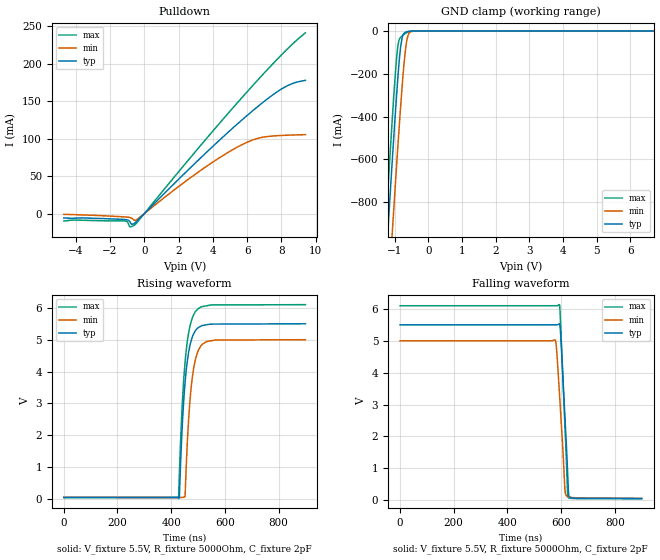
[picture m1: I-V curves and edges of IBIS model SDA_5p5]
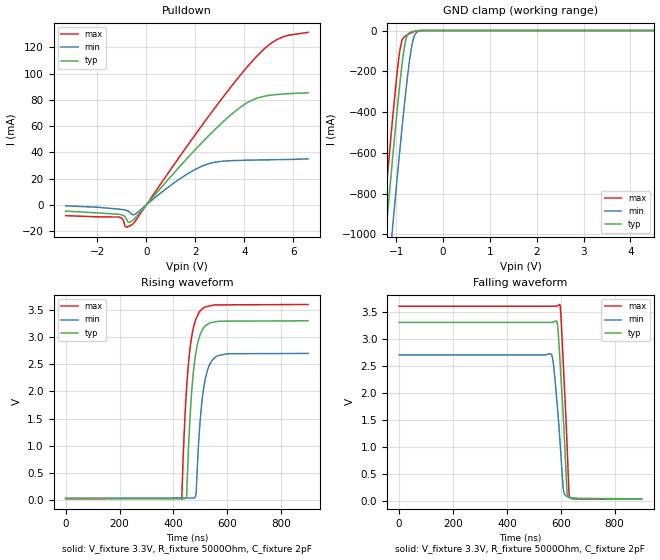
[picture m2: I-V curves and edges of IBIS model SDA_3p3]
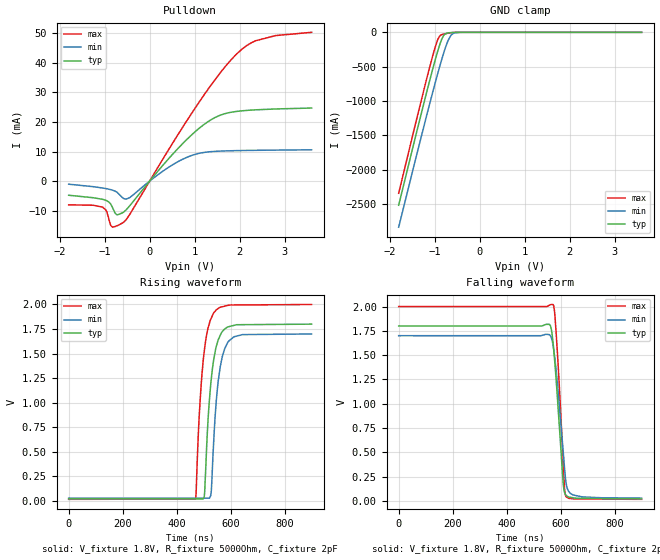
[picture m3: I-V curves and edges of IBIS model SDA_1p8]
[IBIS Ver]   4.1
[File name]   tmp4719.ibs
[File Rev]   1.0
[Date]   07/26/2024
[Source]
| Texas Instruments Incorporated.
| 12500 TI Blvd
| Dallas, TX -75243
[Notes]   Revision History:
| Rev 1.0: 07/29/2024
| - Initial version of the model
| - Model generated from simulations in TISPICE
| - C_comp although listed in numerical order of value are
|   obtained from varying PVT conditions. For PVT conditions for
|   each specific value refer the buffer description under
|   respective [Model]. IBIS model user is responsible for using
|   appropriate C_comp to simulate for Signal Integrity.
| - Warnings regarding combined Non-monotonicity of various models have been
|   reviewd and considered minor and can be ignored.
| - Model names with a trailing _1p8 contains the model for
|   1.8V operation. Model names with a trailing _3p3 contains the model
|   for 3.3V operation. Model names with a trailing _5p5 contains the model
|   for 5.5V operation.
[Disclaimer]
| This model is designed as an aid for customers of Texas Instruments.
| TI and its licensors and suppliers make no warranties, either expressed
| or implied, with respect to this  model, including the warranties of
| merchantability or fitness for a particular purpose. The model is
| provided solely on an "as is" basis. The entire risk as to its quality
| and performance is with the customer.
[Copyright]
 (C) Copyright 2024 Texas Instruments Incorporated.All rights reserved.
|   Device
[Component]   TMP4719
[Manufacturer]   TI
[Package]   |DGK 10 pin
| variable   typ   min   max
R_pkg   0.083   0.076   0.088
L_pkg   1.774nH   1.670nH   1.869nH
C_pkg   0.393pF   0.385pF   0.402pF
[Pin]  signal_name   model_name   R_pin   L_pin   C_pin
1   SDA   SDA   0.08836   1.8688nH   0.38537pF
2   SCL   SCL   0.0798   1.72452nH   0.40219pF
3   ALERT   ALERT   0.07626   1.67019nH   0.40077pF
4   T_CRIT   T_CRIT   0.07626   1.67019nH   0.40077pF
5   GND   GND   0.08804   1.86388nH   0.38801pF
6   V+   POWER   0.08723   1.84409nH   0.38521pF
|   Model Selectors
[Model Selector]  SDA
SDA_5p5  SDA buffer at 5.5V operation.
SDA_3p3  SDA buffer at 3.3V operation.
SDA_1p8  SDA buffer at 1.8V operation.
[Model Selector]  SCL
SCL_5p5  SCL buffer at 5.5V operation.
SCL_3p3  SCL buffer at 3.3V operation.
SCL_1p8  SCL buffer at 1.8V operation.
[Model Selector]  T_CRIT
T_CRIT_5p5  TCRIT buffer at 5.5V operation.
T_CRIT_3p3  TCRIT buffer at 3.3V operation.
T_CRIT_1p8  TCRIT buffer at 1.8V operation.
[Model Selector]  ALERT
ALERT_5p5  ALERT buffer at 5.5V operation.
ALERT_3p3  ALERT buffer at 3.3V operation.
ALERT_1p8  ALERT buffer at 1.8V operation.
| Models and submodels in the file (12): SDA_5p5 (I/O_open_drain), SDA_3p3 (I/O_open_drain), SDA_1p8 (I/O_open_drain), SCL_5p5 (Input), SCL_3p3 (Input), SCL_1p8 (Input), T_CRIT_5p5 (Open_drain), T_CRIT_3p3 (Open_drain), T_CRIT_1p8 (Open_drain), ALERT_5p5 (Open_drain), ALERT_3p3 (Open_drain), ALERT_1p8 (Open_drain)
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|   Model
[Model]   SDA_5p5
Model_type   I/O_open_drain
Polarity   Non-Inverting
Enable   Active-Low
Vinl = .4
Vinh = .9
Vmeas = 2.75
Vref = 5.5
Cref = 2pF
Rref = 5000
|   typ   min   max
C_comp   1.53pF   1.52pF   1.55pF
[Voltage Range]   5.5   5   6.1
[Temperature Range]   25   125   -40
[Pullup Reference]   5.5   5   6.1
[Pulldown Reference]   0   -0   -0
[Power Clamp Reference]   5.5   5   6.1
[GND Clamp Reference]   0   0   0
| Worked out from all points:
|   slope of the pulldown table from 0 to 0.825 V, typ, clamps not added: 43.3 ohm
|   GND clamp passes 1 mA (typ) near -0.56 V on its own axis
|   falling waveform, V_fixture 5.5V, R_fixture 5000Ohm, C_fixture 2pF: 20-80 % time 19.6ns typ, 21ns min, 18.3ns max; typ from 5.5 V to 0.048 V
|   rising waveform, V_fixture 5.5V, R_fixture 5000Ohm, C_fixture 2pF: 20-80 % time 26.3ns typ, 25.8ns min, 26.7ns max; typ from 0.048 V to 5.5 V
[Pulldown]
-4.7V     -5.81mA    -1.013mA   -9.912mA
-1.175V   -7.78mA    -4.349mA   -9.649mA
-977.6mV  -8.471mA   -4.734mA   -11.18mA
-836.6mV  -10.98mA   -5.246mA   -17.65mA
-709.7mV  -14.3mA    -6.455mA   -16.85mA
-568.7mV  -12.77mA   -8.943mA   -15.24mA
3.267V    73.81mA    57.22mA    90.31mA
5.734V    125.6mA    92.29mA    155.6mA
6.763V    145.4mA    101.2mA    181.6mA
8.004V    166.1mA    104.2mA    211.6mA
8.681V    173.7mA    104.8mA    226.8mA
9.4V      177.6mA    105.3mA    241mA
[GND Clamp]
|   Voltage   I(typ)   I(min)   I(max)
-4.7V     -10.05A    -9.956A    -10.16A
-1.429V   -1.526A    -1.858A    -1.339A
-1.175V   -864.5mA   -1.203A    -669.8mA
-1.062V   -580.7mA   -918.6mA   -386.8mA
-963.5mV  -344.9mA   -676.4mA   -164.1mA
-893mV    -192mA     -509.3mA   -57.85mA
-822.5mV  -71.81mA   -350.5mA   -29.37mA
-780.2mV  -31.43mA   -261.5mA   -23.09mA
-667.4mV  -5.295mA   -71.65mA   -9.38mA
-582.8mV  -1.501mA   -12.63mA   -2.903mA
-441.8mV  -35.9uA    -371.1uA   -36.31uA
9.4V      0A         0A         0A
[Ramp]
R_load = 5000
|   typ   min   max
dV/dt_r   3.27126/2.62432e-08   2.96756/2.58579e-08   3.63356/2.67118e-08
dV/dt_f   3.27121/1.95677e-08   2.96741/2.09694e-08   3.63356/1.82625e-08
[Falling Waveform]
V_fixture = 5.5V
V_fixture_min = 5V
V_fixture_max = 6.1V
R_fixture = 5000Ohm
C_fixture = 2pF
|   Time   V(typ)   V(min)   V(max)
0s        5.5V       5V         6.1V
577.5ns   5.5V       5.025V     6.1V
582.9ns   5.5V       4.745V     6.1V
593.5ns   5.533V     3.377V     6.134V
598.4ns   5.165V     2.705V     5.456V
614.3ns   2.578V     325.8mV    2.311V
625.8ns   519.7mV    102.1mV    91.43mV
628.9ns   141.5mV    91.63mV    65.89mV
637.4ns   70.73mV    82.72mV    54.57mV
900ns     47.98mV    54.31mV    44.06mV
[Rising Waveform]
V_fixture = 5.5V
V_fixture_min = 5V
V_fixture_max = 6.1V
R_fixture = 5000Ohm
C_fixture = 2pF
|   Time   V(typ)   V(min)   V(max)
0s        47.85mV    53.99mV    44.02mV
427.5ns   54.74mV    49.34mV    10.99mV
430.4ns   38.26mV    49.31mV    744.4mV
439.6ns   2.002V     49.21mV    2.679V
451.8ns   3.655V     109.9mV    4.292V
460ns     4.313V     1.743V     4.933V
468.3ns   4.754V     2.904V     5.361V
488.9ns   5.263V     4.324V     5.862V
531.8ns   5.47V      4.941V     6.065V
900ns     5.5V       5V         6.1V
|   Model
[Model]   SDA_3p3
Model_type   I/O_open_drain
Polarity   Non-Inverting
Enable   Active-Low
Vinl = .4
Vinh = .9
Vmeas = 1.65
Vref = 3.3
Cref = 2pF
Rref = 5000
|   typ   min   max
C_comp   1.69pF   1.64pF   1.76pF
[Voltage Range]   3.3   2.7   3.6
[Temperature Range]   25   125   -40
[Pullup Reference]   3.3   2.7   3.6
[Pulldown Reference]   0   -0   -0
[Power Clamp Reference]   3.3   2.7   3.6
[GND Clamp Reference]   0   0   0
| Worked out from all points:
|   slope of the pulldown table from 0 to 0.495 V, typ, clamps not added: 45.8 ohm
|   GND clamp passes 1 mA (typ) near -0.56 V on its own axis
|   falling waveform, V_fixture 3.3V, R_fixture 5000Ohm, C_fixture 2pF: 20-80 % time 21.4ns typ, 24.3ns min, 19.7ns max; typ from 3.3 V to 0.03 V
|   rising waveform, V_fixture 3.3V, R_fixture 5000Ohm, C_fixture 2pF: 20-80 % time 27.6ns typ, 27.5ns min, 28.2ns max; typ from 0.03 V to 3.3 V
[Pulldown]
|   Voltage   I(typ)   I(min)   I(max)
-3.3V     -4.897mA   -798.3uA   -8.335mA
-1.132V   -7.293mA   -3.329mA   -9.384mA
-973.5mV  -7.926mA   -3.697mA   -10.88mA
-815.1mV  -11.16mA   -4.318mA   -17.1mA
-726mV    -13.47mA   -5.063mA   -16.49mA
-577.5mV  -12.23mA   -7.515mA   -14.98mA
2.095V    44.04mA    27.89mA    56.09mA
2.788V    57.21mA    32.4mA     73.71mA
3.897V    75.21mA    33.87mA    100.3mA
4.511V    81.29mA    34.12mA    113.4mA
5.283V    83.98mA    34.34mA    125.5mA
6.6V      85.38mA    34.99mA    131.5mA
[GND Clamp]
|   Voltage   I(typ)   I(min)   I(max)
-3.3V     -6.595A    -6.844A    -6.468A
-1.35V    -1.318A    -1.652A    -1.128A
-1.201V   -931.7mA   -1.27A     -737.4mA
-1.073V   -606.2mA   -944.3mA   -411.9mA
-924mV    -256.8mA   -582mA     -94.25mA
-874.5mV  -155.9mA   -466.7mA   -44.89mA
-815.1mV  -62.76mA   -334.5mA   -28.17mA
-765.6mV  -23.44mA   -232.3mA   -21.06mA
-696.3mV  -7.668mA   -110.2mA   -12.39mA
-597.3mV  -1.937mA   -17.69mA   -3.745mA
-448.8mV  -45.19uA   -447.2uA   -48.63uA
6.6V      0A         0A         0A
[Ramp]
R_load = 5000
|   typ   min   max
dV/dt_r   1.96185/2.76586e-08   1.59954/2.7379e-08   2.14403/2.82479e-08
dV/dt_f   1.96179/2.14072e-08   1.59935/2.42408e-08   2.14403/1.96887e-08
[Falling Waveform]
V_fixture = 3.3V
V_fixture_min = 2.7V
V_fixture_max = 3.6V
R_fixture = 5000Ohm
C_fixture = 2pF
|   Time   V(typ)   V(min)   V(max)
0s        3.3V       2.7V       3.6V
562.8ns   3.3V       2.718V     3.6V
571.7ns   3.305V     2.562V     3.6V
585.8ns   3.31V      1.827V     3.606V
595.7ns   2.701V     1.192V     3.631V
599.6ns   2.367V     899.7mV    3.495V
609.6ns   1.518V     215.2mV    2.502V
623ns     173.6mV    79.91mV    1.066V
632.9ns   57.26mV    62.87mV    65.42mV
900ns     30.34mV    34.42mV    26.62mV
[Rising Waveform]
V_fixture = 3.3V
V_fixture_min = 2.7V
V_fixture_max = 3.6V
R_fixture = 5000Ohm
C_fixture = 2pF
|   Time   V(typ)   V(min)   V(max)
0s        30.19mV    34mV       26.56mV
430.9ns   27.19mV    38.85mV    14.82mV
448.7ns   42.53mV    39.05mV    2.048V
455.8ns   940.7mV    39.13mV    2.51V
469.1ns   2.079V     39.28mV    3.045V
484.1ns   2.737V     113.7mV    3.341V
494.7ns   2.97V      1.141V     3.453V
517.7ns   3.203V     2.217V     3.555V
554ns     3.28V      2.626V     3.593V
900ns     3.3V       2.7V       3.6V
|   Model
[Model]   SDA_1p8
Model_type   I/O_open_drain
Polarity   Non-Inverting
Enable   Active-Low
Vinl = .4
Vinh = .9
Vmeas = 0.9
Vref = 1.8
Cref = 2pF
Rref = 5000
|   typ   min   max
C_comp   5pF   5pF   5pF
[Voltage Range]   1.8   1.7   2
[Temperature Range]   25   125   -40
[Pullup Reference]   1.8   1.7   2
[Pulldown Reference]   0   0   -0
[Power Clamp Reference]   1.8   1.7   2
[GND Clamp Reference]   0   0   0
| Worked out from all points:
|   slope of the pulldown table from 0 to 0.27 V, typ, clamps not added: 54.9 ohm
|   GND clamp passes 1 mA (typ) near -0.55 V on its own axis
|   falling waveform, V_fixture 1.8V, R_fixture 5000Ohm, C_fixture 2pF: 20-80 % time 26.7ns typ, 31.2ns min, 22.8ns max; typ from 1.8 V to 0.02 V
|   rising waveform, V_fixture 1.8V, R_fixture 5000Ohm, C_fixture 2pF: 20-80 % time 29.1ns typ, 28.6ns min, 29.6ns max; typ from 0.019 V to 1.8 V
[Pulldown]
|   Voltage   I(typ)   I(min)   I(max)
-1.8V     -4.782mA   -1.047mA   -8.032mA
-1.049V   -6.151mA   -2.332mA   -8.796mA
-957.6mV  -6.625mA   -2.576mA   -10.19mA
-828mV    -8.868mA   -3.058mA   -15.57mA
-730.8mV  -11.37mA   -3.725mA   -15.15mA
-595.8mV  -10.68mA   -5.713mA   -14.1mA
-444.6mV  -8.385mA   -5.604mA   -11.33mA
991.8mV   16.43mA    8.955mA    24.25mA
1.445V    21.44mA    10.04mA    34.15mA
1.899V    23.5mA     10.29mA    42.45mA
2.353V    24.1mA     10.41mA    47.45mA
3.6V      24.71mA    10.58mA    50.32mA
[GND Clamp]
|   Voltage   I(typ)   I(min)   I(max)
-1.8V     -2.517A    -2.836A    -2.342A
-1.195V   -916.3mA   -1.254A    -721.9mA
-984.6mV  -393.8mA   -727.5mA   -207.9mA
-936mV    -283mA     -610.5mA   -113.1mA
-892.8mV  -191.6mA   -508.9mA   -57.68mA
-806.4mV  -53.2mA    -315.9mA   -26.85mA
-752.4mV  -18.22mA   -206.7mA   -19.27mA
-703.8mV  -8.474mA   -121.6mA   -13.23mA
-633.6mV  -3.381mA   -38.72mA   -6.354mA
-568.8mV  -1.148mA   -9.045mA   -2.206mA
-439.2mV  -32.98uA   -346.1uA   -32.57uA
3.6V      0A         0A         0A
[Ramp]
R_load = 5000
|   typ   min   max
dV/dt_r   1.06834/2.90779e-08   1.00319/2.8609e-08   1.19049/2.96432e-08
dV/dt_f   1.06826/2.6653e-08   1.00284/3.119e-08   1.19048/2.28048e-08
[Falling Waveform]
V_fixture = 1.8V
V_fixture_min = 1.7V
V_fixture_max = 2V
R_fixture = 5000Ohm
C_fixture = 2pF
|   Time   V(typ)   V(min)   V(max)
0s        1.8V       1.7V       2V
558.4ns   1.817V     1.711V     2.013V
572.1ns   1.623V     1.599V     2.021V
577.9ns   1.445V     1.482V     1.935V
584.5ns   1.205V     1.312V     1.682V
609.1ns   194.2mV    522.1mV    413mV
614.7ns   86.7mV     329mV      121.2mV
619ns     61.67mV    209.6mV    49.96mV
647ns     31.62mV    60.13mV    21.23mV
900ns     19.57mV    28.59mV    15.87mV
[Rising Waveform]
V_fixture = 1.8V
V_fixture_min = 1.7V
V_fixture_max = 2V
R_fixture = 5000Ohm
C_fixture = 2pF
|   Time   V(typ)   V(min)   V(max)
0s        19.37mV    27.91mV    15.8mV
467.9ns   20.2mV     27.31mV    18.41mV
472.3ns   20.21mV    27.31mV    87.5mV
487.6ns   20.23mV    27.29mV    1.047V
502.6ns   49.77mV    27.27mV    1.528V
526ns     1.179V     53.23mV    1.847V
535.8ns   1.411V     526.9mV    1.907V
561.3ns   1.685V     1.363V     1.972V
593.4ns   1.774V     1.629V     1.993V
900ns     1.8V       1.7V       2V
